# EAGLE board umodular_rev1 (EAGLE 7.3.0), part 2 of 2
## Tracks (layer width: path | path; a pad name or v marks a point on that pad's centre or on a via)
GND  (via drill 0.51)
  Top 0.356: 5K1.3 90.27,89.97 90.27,92.71 88.14,94.84 5K1.2 | 102.77,71.07 102.77,68.33 10K1.2 | 102.77,71.07 104.9,73.2 10K1.1 | 102.77,71.07 100.02,71.07 93.32,77.77 R18.P$1 | R15.P$2 82.96,84.18 86.92,84.18 93.02,78.08 R18.P$1 | TL274.10 75.95,40.89 77.77,42.72 77.77,43.94 75.95,45.77 TL274.12 | 10K.1 63.45,71.07 63.45,68.33 10K.2 63.14,68.33 61.01,66.19 61.01,65.28 64.06,62.23 64.06,50.04 68.02,46.08 TL274.3 | CA3046.4 75.95,63.45 77.77,63.45 82.65,68.33 R17.P$1 82.96,68.33 92.41,77.77 93.02,77.77 R18.P$1 | 197.87,69.85 198.48,69.85 199.39,70.76 DUALOPAMP.3 | 197.87,69.85 192.99,69.85 TL274-6.10 192.68,69.85 185.37,69.85 TL274-6.5 | 197.87,69.85 197.87,64.06 R99.P$1 | LM13700.13 161.9,83.26 165.25,83.26 166.17,84.18 C11.2 166.47,84.48 169.22,84.48 C10.2 | R56.P$1 175.31,87.22 178.66,83.87 181.1,83.87 R93.P$1 181.41,83.87 182.93,83.87 186.28,87.22 THAT2180.3 186.59,87.22 188.42,85.39 192.08,85.39 193.9,87.22 THAT2180.6 194.21,87.53 196.65,89.97 202.74,89.97 210.36,97.59 236.27,97.59 237.8,96.06 D1.A 238.1,95.76 239.32,94.54 241.45,94.54 244.5,91.49 | RES0NANCE.P$1 141.48,37.54 141.48,53.7 139.34,55.83 139.34,67.41 R48.P$2 139.04,67.72 139.04,69.24 135.99,72.29 135.99,78.08 | TL274-3.10 115.27,40.89 117.09,42.72 117.09,43.94 115.27,45.77 TL274-3.12 | R31.P$1 102.16,40.59 107.34,45.77 TL274-3.3 | CA3046-2.4 115.57,63.45 117.4,63.45 122.28,68.33 R40.P$1 122.58,68.33 132.33,78.08 | 5K3.3 129.9,89.97 129.9,92.41 127.46,94.84 5K3.2 | 135.99,78.08 132.64,78.08 R41.P$1 132.33,78.08 | R55.P$1 135.99,78.08 | 132.33,78.08 126.24,84.18 122.58,84.18 R38.P$2
  Top 0.356: U2.SLEEVE 368.86,17.12 368.86,18.03 372.52,21.69 372.52,43.64 368.86,47.3 U1.SLEEVE | 320.4,37.85 322.22,36.02 TL274-8.5 322.53,36.02 326.19,36.02 328.02,37.85 | 320.4,37.85 320.4,39.07 322.22,40.89 TL274-8.3 | 328.02,37.85 329.84,36.02 TL274-8.10 | 328.02,37.85 328.02,39.07 329.84,40.89 TL274-8.12 | 293.27,10.41 293.27,9.8 C17.1 | 293.27,10.41 289.92,13.77 ATT1.P$1 289.61,13.77 284.12,13.77 275.89,5.54 275.89,4.01 274.98,3.1 269.19,3.1 262.79,9.5 249.38,9.5 C14.1 249.07,9.8 244.5,14.38 ATT.P$1 244.5,14.68 244.5,17.73 251.82,25.04 251.82,33.27 C13.1 | 293.27,10.41 296.32,13.46 296.32,18.64 294.79,20.17 294.79,30.84 296.62,32.66 C16.1 296.93,32.97 301.8,37.85 320.4,37.85 | 555-1.1 288.7,86.31 288.7,96.06 287.17,97.59 284.43,97.59 282.9,96.06 D6.A 282.6,96.06 281.69,96.06 280.16,97.59 250.6,97.59 244.5,91.49 | 2N3904-4.1 276.2,70.46 276.2,75.95 2N3904-1.1 | v276.81,67.41 276.81,61.62 2N3904-5.1 | 244.5,91.49 244.5,86.61 | 244.5,86.61 244.5,86.31 555.1 244.5,86.61 | 2N3904.1 232,61.62 232,69.55 231.39,70.16 2N3904-2.1 231.39,70.46 231.39,74.42 | 231.39,74.42 231.39,75.95 2N3904-3.1 | 244.5,86.61 239.62,86.61 237.49,84.48 237.49,76.86 237.8,76.56 237.8,75.34 236.88,74.42 231.39,74.42
  Bottom 0.356: 5K1.3 90.58,89.66 90.58,80.52 93.02,78.08 R18.P$1 | R8.P$1 62.54,40.59 61.01,42.11 61.01,50.04 56.74,54.3 JP3.2 56.74,54.61 61.01,58.88 61.01,66.19 63.14,68.33 10K.2 | TL274.3 68.33,45.77 75.64,45.77 TL274.12 | 10K.1 65.89,73.2 68.33,73.2 73.81,67.72 73.81,65.58 75.95,63.45 CA3046.4 | TL274-6.5 185.37,69.85 187.2,71.68 187.2,72.9 185.37,74.73 TL274-6.3 | R56.P$1 175.01,87.22 172.26,87.22 169.52,84.48 C10.2 | DUALOPAMP.3 199.39,71.07 199.39,71.68 194.82,76.25 194.82,86.61 194.21,87.22 THAT2180.6 | TL274-3.12 114.96,45.77 107.64,45.77 TL274-3.3 107.34,46.08 105.51,47.9 105.51,51.26 108.56,54.3 108.86,54.3 113.44,58.88 113.44,61.32 115.27,63.14 CA3046-2.4 115.27,63.45 113.44,65.28 113.44,67.72 107.95,73.2 105.21,73.2 10K1.1 | R41.P$1 132.33,78.08 130.2,80.21 130.2,89.66 5K3.3 130.2,89.97 132.94,92.71 149.71,92.71 152.76,89.66 155.19,89.66 161.59,83.26 LM13700.13 | C16.1 296.62,32.97 296.62,36.02 292.35,40.28 292.35,48.51 289.31,51.56 D7.A | U2.SLEEVE 368.55,16.81 368.55,14.38 364.29,10.11 361.24,10.11 336.55,34.8 336.55,38.76 334.42,40.89 330.15,40.89 TL274-8.12 | v276.81,67.41 276.81,69.85 276.5,70.16 2N3904-4.1 | D6.A 282.6,95.76 282.6,93.02 276.5,86.92 276.5,76.25 2N3904-1.1 | 2N3904.1 232.31,61.62 242.06,51.87 D2.A 244.5,51.56 244.5,32.97 245.42,32.05 246.63,32.05 247.85,33.27 251.82,33.27 C13.1
  pour Bottom: 0.1,99.85 373.28,99.85 373.28,0 0.1,0
N$1
  Top 0.356: R6.P$2 R5.P$2 | R2.P$2 62.84,27.79 65.58,27.79 R3.P$2 65.89,27.79 68.94,27.79 R4.P$2
  Bottom 0.356: TL274.2 68.02,48.21 62.84,43.03 R1.P$1 62.84,42.72 62.84,42.11 65.58,39.37 65.58,27.79 R3.P$2 | R6.P$2 65.58,14.99 65.58,15.6 64.06,17.12 64.06,26.26 62.84,27.48 R2.P$2
N$2
  Bottom 0.356: R1.P$2 62.84,53.09 64.97,50.95 68.02,50.95 TL274.1 68.33,50.65 71.98,46.99 77.16,46.99 80.82,43.33 83.26,43.33 87.83,38.76 93.02,38.76 R7.P$2
N$3
  Top 0.356: CVS.5 79.6,21.08 66.19,21.08 62.84,17.73 R2.P$1
N$4
  Top 0.356: CVS.4 79.91,18.95 67.11,18.95 65.89,17.73 R3.P$1
N$5
  Top 0.356: CVS.3 79.6,16.51 70.16,16.51 69.24,17.42 R4.P$1
N$6
  Top 0.356: CVS.2 79.91,13.46 71.37,13.46 62.84,4.93 R5.P$1
N$7
  Top 0.356: R6.P$1 71.98,11.02 79.6,11.02 CVS.1
N$8
  Top 0.356: R7.P$1 82.96,38.46 82.96,31.75 83.57,31.14 5K.3
N$9
  Top 0.356: 5K.1 78.69,31.14 78.69,33.58 80.82,35.71 5K.2 | TL274.5 68.02,40.59 62.84,35.41 62.84,30.23 R8.P$2
  Bottom 0.356: 5K.1 78.38,31.14 77.77,31.14 68.33,40.59 TL274.5
N$10
  Top 0.356: TL274.7 68.33,35.71 68.33,38.15 TL274.6 68.33,38.46 70.16,40.28 70.16,52.17 75.95,57.96 CA3046.2
N$11
  Top 0.356: JP1.3 93.02,21.39 93.02,34.49 82.96,44.55 R11.P$1
N$12
  Top 0.356: TL274.8 75.95,35.71 78.38,38.15 78.38,48.51 79.6,49.73 C1.2 79.91,50.04 81.43,51.56 82.65,51.56 R10.P$1
N$13
  Top 0.356: CA3046.5 75.95,65.89 77.16,65.89 82.65,71.37 R12.P$1
N$14
  Top 0.356: CA3046.1 75.95,55.52 72.29,51.87 72.29,41.81 75.64,38.46 TL274.9 75.64,38.15 73.81,36.32 73.81,35.1 74.73,34.19 76.86,34.19 79.6,36.93 79.6,47.3 C1.1
  Bottom 0.356: 91.49,46.38 82.96,46.38 82.04,47.3 79.91,47.3 C1.1 | 91.49,46.38 93.02,44.86 R11.P$2 | 91.49,46.38 91.49,52.17 93.02,53.7 93.02,54.91 R9.P$1
N$15
  Top 0.356: CA3046.3 84.18,60.71 93.02,51.87 R10.P$2
N$16
  Top 0.356: C2.1 82.65,63.14 85.09,60.71 87.53,60.71 J112.2 87.83,60.71 87.83,65.28 93.02,70.46 93.02,71.37 R12.P$2
  Bottom 0.356: TL274.13 75.95,48.51 80.21,52.78 80.21,61.01 82.35,63.14 C2.1
N$17
  Top 0.356: C4.1 79.3,72.29 80.52,72.29 82.65,74.42 R13.P$1 | TL274.14 75.95,50.95 75.95,51.87 82.35,58.27 C2.2
  Bottom 0.356: C2.2 82.65,58.57 83.26,59.18 89.36,59.18 J112.3 89.66,59.49 90.88,60.71 90.88,65.58 82.96,73.51 82.96,74.42 R13.P$1
N$18
  Top 0.356: TL274-2.10 68.02,86 65.28,86 64.67,86.61 R20.P$2
N$19
  Top 0.356: C3.2 78.99,77.16 77.47,77.16 75.95,75.64 TL274-2.1
  Bottom 0.356: J112.1 89.36,62.23 86.92,62.23 75.95,73.2 75.95,75.34 TL274-2.1
N$20
  Top 0.356: TL274-2.9 68.33,88.14 73.81,82.65 73.81,60.4 74.73,59.49 81.43,59.49 81.74,59.79 82.96,59.79 93.02,49.73 93.02,48.82 R21.P$1
N$21
  Top 0.356: R15.P$1 93.32,84.18 93.32,81.13 R14.P$2
  Bottom 0.356: TL274-2.2 75.95,78.08 78.08,75.95 82.04,75.95 82.35,76.25 89.36,76.25 92.41,73.2 93.62,73.2 94.54,74.12 94.54,79.6 93.32,80.82 R14.P$2
N$22
  Top 0.356: JP1.1 93.02,16.51 85.09,24.43 85.09,41.5 83.26,43.33 82.35,43.33 81.43,44.25 81.43,47.3 82.65,48.51 R21.P$2
N$23
  Top 0.356: TL274-2.3 75.95,80.52 78.38,80.52 78.99,79.91 C3.1 | 93.32,68.33 94.54,67.11 94.54,44.25 93.32,43.03 93.32,41.81 R16.P$1 | 93.32,68.33 94.54,69.55 94.54,72.29 93.32,73.51 93.32,74.42 R13.P$2 | 93.32,68.33 R17.P$2
  Bottom 0.356: C3.1 79.3,79.6 88.14,79.6 93.02,74.73 R13.P$2
N$24
  Bottom 0.356: JP1.2 93.32,18.95 92.71,18.95 85.09,26.57 85.09,39.37 82.96,41.5 R16.P$2
N$25
  Top 0.356: 82.65,78.08 82.65,78.99 75.95,85.7 TL274-2.5 | 82.65,78.08 79.3,74.73 C4.2 | 82.65,78.08 R18.P$2
N$26
  Top 0.356: TL274-2.6 75.95,88.44 82.04,88.44 83.26,89.66 85.39,89.66 5K1.1 85.7,89.66 87.83,87.53 93.02,87.53 R19.P$1
N$27
  Top 0.356: JP2.2 93.02,7.06 93.02,10.72 77.47,26.26 61.93,26.26 53.39,34.8 53.39,64.06 64.36,75.03 64.36,76.56 R20.P$1
  Bottom 0.356: R19.P$2 82.65,87.53 79.6,90.58 75.95,90.58 TL274-2.7 75.64,90.58 69.55,84.48 66.8,84.48 64.67,82.35 64.67,76.86 R20.P$1
N$28
  Top 0.356: TL274-2.8 68.02,90.58 61.62,90.58 R22.P$1
N$29
  Top 0.356: R22.P$2 61.32,80.21 61.32,74.12 60.71,73.51 10K.3
  Bottom 0.356: JP2.1 93.02,4.32 92.1,4.32 81.43,14.99 76.25,14.99 64.06,27.18 64.06,36.93 54,46.99 54,66.5 60.71,73.2 10K.3
N$30
  Top 0.356: TL274-3.2 107.34,48.21 102.16,43.03 R24.P$1 | R29.P$2 R28.P$2 | R25.P$2 102.16,27.79 104.9,27.79 R26.P$2 105.21,27.79 108.25,27.79 R27.P$2
  Bottom 0.356: R29.P$2 104.9,14.99 104.9,15.6 103.38,17.12 103.38,26.26 102.16,27.48 R25.P$2 | R24.P$1 102.16,42.72 104.9,39.98 104.9,27.79 R26.P$2
N$31
  Top 0.356: CA3046.14 CA3046.13 CA3046.12 63.45,65.58 62.84,65.58 R23.P$2
N$32
  Top 0.356: TL274-3.1 107.34,50.95 104.29,50.95 102.16,53.09 R24.P$2
  Bottom 0.356: R30.P$2 132.33,38.76 127.15,38.76 122.58,43.33 120.14,43.33 116.48,46.99 111.3,46.99 107.64,50.65 TL274-3.1
N$33
  Top 0.356: CVS1.5 118.92,21.08 105.51,21.08 102.16,17.73 R25.P$1
N$34
  Top 0.356: CVS1.4 119.23,18.95 106.43,18.95 105.21,17.73 R26.P$1
N$35
  Top 0.356: CVS1.3 118.92,16.51 109.47,16.51 108.56,17.42 R27.P$1
N$36
  Top 0.356: CVS1.2 119.23,13.46 110.69,13.46 102.16,4.93 R28.P$1
N$37
  Top 0.356: CVS1.1 118.92,11.02 111.3,11.02 105.21,4.93 R29.P$1
N$38
  Top 0.356: R30.P$1 122.58,38.46 122.58,31.45 122.88,31.14 5K2.3
N$39
  Top 0.356: 5K2.1 118.01,31.14 118.01,33.58 120.14,35.71 5K2.2 | TL274-3.5 107.34,40.59 102.16,35.41 102.16,30.23 R31.P$2
  Bottom 0.356: 5K2.1 117.7,31.14 117.09,31.14 107.64,40.59 TL274-3.5
N$40
  Top 0.356: 107.64,38.15 107.64,35.71 TL274-3.7 | 107.64,38.15 109.47,39.98 109.47,52.17 115.27,57.96 CA3046-2.2 | 107.64,38.15 TL274-3.6
N$41
  Top 0.356: TL274-3.8 115.27,35.71 117.7,38.15 117.7,48.51 118.92,49.73 C5.2 119.23,50.04 120.75,51.56 122.28,51.56 R33.P$1
N$42
  Top 0.356: 113.74,38.46 114.96,38.46 TL274-3.9 | 113.74,38.46 110.39,41.81 110.39,50.65 115.27,55.52 CA3046-2.1 | R34.P$2 132.33,44.86 130.81,46.38 122.58,46.38 121.67,47.3 119.23,47.3 C5.1 118.92,47.3 118.92,36.93 116.18,34.19 114.05,34.19 113.13,35.1 113.13,36.02 113.74,36.63 113.74,38.46
  Bottom 0.356: R32.P$1 132.64,54.91 132.64,53.7 133.86,52.48 133.86,46.08 132.64,44.86 R34.P$2
N$43
  Top 0.356: CA3046-2.3 123.49,60.71 132.33,51.87 R33.P$2
N$44
  Top 0.356: R34.P$1 132.33,34.8 132.33,21.39 JP4.3
N$45
  Top 0.356: CA3046-2.5 115.57,65.89 116.79,65.89 122.28,71.37 R35.P$1
N$46
  Top 0.356: C6.1 121.97,63.14 124.41,60.71 126.85,60.71 Q2.2 127.15,60.71 127.15,64.97 132.33,70.16 132.33,71.37 R35.P$2
  Bottom 0.356: TL274-3.13 115.27,48.51 119.84,53.09 119.84,61.32 121.67,63.14 C6.1
N$47
  Top 0.356: C8.1 118.62,72.29 120.14,72.29 122.28,74.42 R36.P$1 | TL274-3.14 115.27,50.95 115.27,51.87 121.67,58.27 C6.2
  Bottom 0.356: C6.2 121.97,58.57 122.58,59.18 128.68,59.18 Q2.3 128.98,59.49 130.2,60.71 130.2,65.58 122.58,73.2 122.58,74.42 R36.P$1
N$48
  Top 0.356: TL274-4.1 115.27,75.64 116.79,75.64 118.31,77.16 C7.2
  Bottom 0.356: Q2.1 128.68,62.23 126.24,62.23 117.4,71.07 117.4,71.37 115.27,73.51 115.27,75.34 TL274-4.1
N$49
  Top 0.356: R38.P$1 132.64,84.18 132.64,81.13 R37.P$2
  Bottom 0.356: TL274-4.2 115.27,78.08 117.4,75.95 121.36,75.95 121.67,76.25 128.68,76.25 131.72,73.2 132.94,73.2 133.86,74.12 133.86,79.6 132.64,80.82 R37.P$2
N$50
  Top 0.356: TL274-4.3 115.27,80.52 117.7,80.52 118.31,79.91 C7.1 | 132.64,68.33 133.86,67.11 133.86,44.25 132.64,43.03 132.64,41.81 R39.P$1 | 132.64,68.33 133.86,69.55 133.86,72.29 132.64,73.51 132.64,74.42 R36.P$2 | 132.64,68.33 R40.P$2
  Bottom 0.356: C7.1 118.62,79.6 127.46,79.6 132.33,74.73 R36.P$2
N$51
  Top 0.356: JP4.2 132.64,18.95 132.03,18.95 124.41,26.57 124.41,39.68 122.58,41.5 R39.P$2
N$52
  Top 0.356: TL274-4.5 115.27,85.7 122.28,78.69 122.28,78.08 R41.P$2 122.28,77.77 119.23,74.73 118.62,74.73 C8.2
N$53
  Top 0.356: TL274-4.6 115.27,88.44 121.36,88.44 122.58,89.66 124.71,89.66 5K3.1 125.02,89.66 127.15,87.53 132.33,87.53 R42.P$1
N$54
  Bottom 0.356: R42.P$2 122.28,87.53 119.23,90.58 115.27,90.58 TL274-4.7 114.96,90.58 108.86,84.48 106.43,84.48 103.99,82.04 103.99,76.86 R43.P$1 103.68,76.56 103.68,75.03 100.33,71.68 100.33,49.73 105.51,44.55 105.51,37.85 106.43,36.93 108.86,36.93 132.33,13.46 132.33,7.06 JP5.2
N$55
  Top 0.356: TL274-4.10 107.34,86 104.6,86 103.99,86.61 R43.P$2
N$56
  Top 0.356: TL274-4.9 107.64,88.14 113.13,82.65 113.13,60.4 114.05,59.49 121.06,59.49 121.36,59.79 122.28,59.79 132.33,49.73 132.33,48.82 R44.P$1
N$57
  Bottom 0.356: JP4.1 132.64,16.51 133.25,16.51 134.77,18.03 134.77,38.15 132.64,40.28 130.81,40.28 122.58,48.51 R44.P$2
N$58
  Top 0.356: TL274-4.8 107.34,90.58 100.94,90.58 R45.P$1
N$59
  Top 0.356: R45.P$2 100.63,80.21 100.63,73.81 100.33,73.51 10K1.3
  Bottom 0.356: JP5.1 132.33,4.32 131.42,4.32 120.75,14.99 115.88,14.99 103.38,27.48 103.38,36.93 99.72,40.59 99.72,72.9 100.02,73.2 10K1.3
N$60
  Top 0.356: CA3046-2.14 107.64,55.83 107.64,57.96 CA3046-2.13 107.64,58.27 107.64,60.71 | 107.64,60.71 102.77,65.58 102.16,65.58 R46.P$2 | 107.64,60.71 CA3046-2.12
N$61
  Top 0.356: C12.2 146.36,63.75 146.36,56.13 145.75,55.52 JP6.1
N$62
  Top 0.356: C12.1 141.48,64.06 141.48,82.04 139.34,84.18 R47.P$1
N$63
  Top 0.356: 156.11,77.47 154.28,75.64 LM13700.7 | 156.11,77.47 156.11,78.69 154.28,80.52 LM13700.5 | 156.11,77.47 156.72,76.86 162.81,76.86 163.73,77.77 163.73,79.3 164.34,79.91 166.17,79.91 168,81.74 169.22,81.74 C10.1
N$64
  Top 0.356: R54.P$1 164.95,78.38 164.95,77.16 163.73,75.95 163.73,75.03 163.12,74.42 159.77,74.42 153.06,67.72 149.4,67.72 R48.P$1
  Bottom 0.356: LM13700.3 153.98,85.7 150.62,85.7 149.4,84.48 R47.P$2 149.4,84.18 150.93,82.65 150.93,70.46 149.4,68.94 149.4,67.72 R48.P$1
N$65
  Top 0.356: LM13700.8 153.98,73.2 150.93,76.25 150.93,78.38 149.4,79.91 146.96,79.91 139.34,87.53 R51.P$2 | JP7.1 174.09,55.22 172.26,53.39 172.26,39.98 174.4,37.85 174.4,36.93 173.18,35.71 148.18,35.71 146.66,37.24 RES0NANCE.P$3 146.36,37.54 146.36,49.73 140.26,55.83 140.26,64.67 140.56,64.97 140.56,75.34 139.34,76.56 139.34,77.77 R50.P$2
  Bottom 0.356: 140.56,86.31 140.56,80.52 139.34,79.3 139.34,78.08 R50.P$2 | 140.56,86.31 139.34,87.53 R51.P$2 | 140.56,86.31 145.14,90.88 149.1,90.88 R49.P$1
N$66
  Top 0.356: R56.P$2 164.95,87.22 163.73,86 161.9,86 LM13700.14 161.59,86 157.94,89.66 148.79,89.66 147.57,90.88 139.34,90.88 R49.P$2
N$67
  Top 0.356: 150.93,82.96 153.98,82.96 LM13700.4 | 150.93,82.96 149.4,81.43 R55.P$2 | 150.93,82.96 150.93,85.09 149.4,86.61 149.4,87.53 R51.P$1
  Bottom 0.356: R53.P$1 149.1,74.73 149.1,76.25 147.88,77.47 147.88,79.91 149.1,81.13 R55.P$2
N$68
  Top 0.356: R53.P$2 139.34,74.42 139.34,71.37 R52.P$2
  Bottom 0.356: R52.P$2 139.34,71.07 141.48,71.07 147.88,64.67 153.37,64.67 161.59,72.9 LM13700.9 161.9,73.2 162.2,73.51 165.25,73.51 166.47,74.73 166.47,79.3 164.95,80.82 164.95,85.09 172.26,92.41 175.62,92.41 176.84,91.19 176.84,54.91 JP7.2
N$69
  Top 0.356: C11.1 166.17,81.74 162.81,81.74 161.9,80.82 LM13700.12
  Bottom 0.356: LM13700.10 161.59,75.64 159.77,77.47 159.77,78.69 161.59,80.52 LM13700.12
N$70
  Top 0.356: R61.P$2 162.81,71.68 164.95,73.81 164.95,75.03 R58.P$1 | LM13700.1 154.28,90.88 161.59,90.88 LM13700.16 161.9,90.88 164.95,90.88 R57.P$1
  Bottom 0.356: R58.P$1 164.95,75.34 164.95,76.56 163.73,77.77 163.73,89.36 164.95,90.58 R57.P$1
N$71
  Bottom 0.356: RES0NANCE.P$2 143.92,37.54 144.53,37.54 157.63,50.65 157.63,53.09 158.55,54 160.99,54 173.18,66.19 173.18,76.56 175.01,78.38 R54.P$2
N$72
  Bottom 0.356: JP8.2 160.07,55.52 160.07,61.32 168,69.24 168,85.09 173.48,90.58 175.01,90.58 R57.P$2
N$73
  Bottom 0.356: JP8.1 160.07,52.78 160.68,52.78 173.79,65.89 173.79,73.81 175.01,75.03 R58.P$2
N$74
  Bottom 0.356: CUTOFF.P$1 168,37.54 168,59.18 175.01,66.19 175.01,71.98 R60.P$2
N$75
  Top 0.356: R59.P$2 162.81,50.04 171.65,41.2 171.65,38.46 172.57,37.54 CUTOFF.P$3
N$76
  Top 0.356: R61.P$1 152.45,69.24 148.79,69.24 147.88,68.33 147.88,59.18 168.3,38.76 168.91,38.76 170.13,37.54 CUTOFF.P$2
N$77
  Top 0.356: TRIG_IN.1 221.34,22 221.34,16.51 S1.1
  Bottom 0.356: R62.P$1 251.82,95.76 243.59,95.76 241.45,93.62 232.31,93.62 228.96,90.27 227.43,90.27 214.94,77.77 214.94,28.7 221.34,22.3 TRIG_IN.1
N$78
  Top 0.356: 2N3904-3.2 233.53,76.25 233.53,92.71 230.48,95.76 D1.C
  Bottom 0.356: D1.C 230.48,95.76 235.97,95.76 237.19,94.54 240.23,94.54 241.45,95.76 R62.P$2
N$79
  Top 0.356: 555.2 244.5,83.87 241.45,83.87 240.23,85.09 R67.P$1
  Bottom 0.356: 2N3904.3 237.19,61.62 237.19,69.24 240.54,72.59 240.54,84.78 240.23,85.09 R67.P$1
N$80
  Top 0.356: 555.4 244.5,78.38 236.58,70.46 2N3904-2.3 | C9.1 251.82,42.72 251.21,42.72 240.54,32.05 239.32,32.05 237.8,33.58 237.8,47.6 239.62,49.43 R70.P$1
  Bottom 0.356: R65.P$1 239.01,88.44 242.67,84.78 242.67,80.52 244.5,78.69 555.4 | 2N3904-2.3 236.27,70.16 236.27,68.02 230.48,62.23 230.48,59.18 239.93,49.73 R70.P$1
N$81
  Top 0.356: 2N3904-3.3 236.58,76.25 236.58,89.97 238.71,92.1 R63.P$1 239.01,92.41 241.45,92.41 R64.P$1
N$82
  Top 0.356: 2N3904-2.2 233.83,70.46 243.28,79.91 246.02,79.91 250.29,84.18 250.29,90.58 251.82,92.1 R64.P$2
N$83
  Top 0.356: D2.C 251.82,51.56 251.82,48.21 C9.2 251.82,47.9 247.55,43.64 246.02,43.64 R66.P$1
N$84
  Bottom 0.356: 2N3904.2 234.75,61.32 237.19,58.88 239.93,58.88 247.55,51.26 247.55,35.1 246.02,33.58 R66.P$2
N$85
  Top 0.356: TL274-5.3 244.5,66.8 243.59,65.89 243.28,65.89 239.32,61.93 239.32,59.49 232.92,53.09 232.92,52.78 231.09,50.95 228.96,50.95 225.6,47.6 225.6,47.3 224.69,46.38 223.16,46.38 221.64,47.9 SUSTAIN.P$2
N$86
  Bottom 0.356: 555.5 252.12,78.38 252.12,74.73 250.29,72.9 250.29,40.28 251.82,38.76 C13.2
N$87
  Top 0.356: 555.7 252.12,83.57 237.8,69.24 237.8,62.84 238.71,61.93 238.71,59.79 232.31,53.39 232.31,53.09 230.78,51.56 227.74,51.56 224.38,48.21 SUSTAIN.P$3
N$88
  Bottom 0.356: SUSTAIN.P$1 219.2,48.21 219.2,50.95 225.6,57.35 228.96,57.35 R68.P$1
N$89
  Top 0.356: TL274-5.1 244.5,71.98 244.5,69.85 TL274-5.2 244.5,69.55 242.67,69.55 239.62,66.5 R69.P$1
N$90
  Top 0.356: DECAY.P$1 219.2,63.75 221.34,63.75 DECAY.P$2 221.64,63.75 224.08,66.19 228.96,66.19 R69.P$2
N$91
  Top 0.356: DECAY.P$3 224.38,63.45 224.38,59.79 230.48,53.7 D3.C
N$92
  Top 0.356: C14.2 244.2,9.8 237.19,9.8 D5.C 237.19,9.5 237.19,4.62 D4.A | D3.A 238.4,53.7 240.84,56.13 240.84,58.27 244.5,61.93 TL274-5.5 244.81,62.23 246.63,64.06 246.63,75.34 252.12,80.82 555.6
  Bottom 0.356: D5.C 237.19,9.8 237.19,14.68 239.93,17.42 239.93,31.45 241.45,32.97 241.45,50.34 238.4,53.39 D3.A
N$93
  Top 0.356: 555.3 244.5,81.13 239.32,81.13 239.01,81.43 R71.P$1
N$94
  Top 0.356: ATTACK.P$1 219.2,79.3 221.34,79.3 ATTACK.P$2 221.64,79.3 223.77,81.43 228.65,81.43 R71.P$2
N$95
  Top 0.356: RELEASE.P$1 219.2,32.05 221.34,32.05 RELEASE.P$2 221.64,32.36 221.64,39.68 229.56,47.6 229.56,49.43 R70.P$2
N$96
  Top 0.356: D4.C 229.26,4.62 229.26,7.67 224.38,12.55 224.38,32.05 RELEASE.P$3
N$97
  Bottom 0.356: D5.A 229.26,9.8 229.26,32.05 228.35,32.97 228.35,54.61 230.78,57.05 230.78,57.96 225.6,63.14 225.6,68.33 224.08,69.85 224.08,78.99 ATTACK.P$3
N$98
  Top 0.356: TL274-5.6 244.5,59.18 244.5,57.05 TL274-5.7 244.5,56.74 244.5,55.22 242.06,52.78 242.06,47.9 239.93,45.77 R72.P$1
N$99
  Top 0.356: ATT.P$2 246.94,14.68 249.07,14.68 ATT.P$3 | TL274-5.10 252.12,61.93 242.67,52.48 242.67,46.38 240.54,44.25 239.32,44.25 238.4,45.16 238.4,46.38 239.93,47.9 240.23,47.9 241.45,49.12 241.45,50.04 240.54,50.95 235.05,50.95 229.87,45.77 R72.P$2
  Bottom 0.356: ATT.P$3 249.38,14.68 249.38,29.01 254.25,33.88 254.25,60.1 252.43,61.93 TL274-5.10
N$100
  Top 0.356: R75.P$1 239.93,33.58 239.93,37.24 R74.P$1 239.93,37.54 239.93,41.2 R73.P$1 239.93,41.5 239.93,42.11 252.12,54.3 252.12,56.74 TL274-5.8 252.12,57.05 252.12,59.18 TL274-5.9
N$101
  Top 0.356: JP9.1 236.58,22 236.58,34.49 229.87,41.2 R73.P$2
N$102
  Top 0.356: JP9.2 236.27,19.56 231.39,24.43 231.39,35.71 229.87,37.24 R74.P$2
N$103
  Top 0.356: JP9.3 235.36,18.03 235.05,18.03 229.87,23.22 229.87,33.27 R75.P$2
N$104
  Top 0.356: TRIG_IN1.1 266.75,22 266.75,16.81 266.45,16.51 S2.1
  Bottom 0.356: R76.P$1 296.62,96.06 288.7,96.06 287.17,97.59 281.08,97.59 273.76,90.27 272.24,90.27 259.13,77.16 259.13,29.92 266.75,22.3 TRIG_IN1.1
N$105
  Top 0.356: 278.94,95.76 281.08,95.76 282.3,94.54 285.34,94.54 286.56,95.76 R76.P$2 | 278.94,95.76 275.28,95.76 D6.C | 278.94,95.76 278.94,76.25 2N3904-1.2
N$106
  Top 0.356: 555-1.2 288.7,83.87 285.34,83.87 284.12,85.09 R81.P$1
  Bottom 0.356: 2N3904-5.3 282.3,61.62 282.3,68.33 286.87,72.9 286.87,81.74 288.7,83.57 555-1.2
N$107
  Top 0.356: 287.17,76.25 281.38,70.46 2N3904-4.3 | 287.17,76.25 288.7,77.77 288.7,78.38 555-1.4 | 287.17,76.25 282.3,81.13 282.3,85.7 283.82,87.22 283.82,88.44 R79.P$1
  Bottom 0.356: R84.P$1 285.04,48.82 286.26,47.6 286.26,35.41 290.52,31.14 296.93,31.14 298.14,32.36 298.14,38.46 296.93,39.68 296.93,42.11 C15.1 296.62,42.42 295.4,43.64 295.4,47.6 289.61,53.39 285.04,53.39 282.9,55.52 282.9,56.74 283.51,57.35 283.51,61.62 287.78,65.89 290.22,65.89 290.83,66.5 290.83,72.59 289,74.42 289,78.38 555-1.4
N$108
  Top 0.356: 2N3904-1.3 281.38,76.25 281.38,89.66 283.82,92.1 R77.P$1 284.12,92.41 286.56,92.41 R78.P$1
N$109
  Bottom 0.356: 2N3904-4.2 278.94,70.46 278.94,71.68 285.65,78.38 285.65,85.39 292.35,92.1 296.62,92.1 R78.P$2
N$110
  Top 0.356: D7.C 296.93,51.56 296.93,47.6 C15.2 296.62,47.3 292.35,43.03 291.13,43.03 R80.P$1
N$111
  Bottom 0.356: 2N3904-5.2 279.55,61.32 279.55,57.96 289.31,48.21 289.31,34.49 290.83,32.97 R80.P$2
N$112
  Top 0.356: 555-1.5 296.62,78.38 296.62,74.42 298.45,72.59 298.45,39.68 296.93,38.15 C16.2
N$113
  Bottom 0.356: 555-1.7 296.32,83.87 291.13,83.87 290.22,84.78 287.48,84.78 286.26,83.57 286.26,73.2 268.88,55.83 268.88,48.21 SUSTAIN1.P$3
N$114
  Top 0.356: SUSTAIN1.P$1 264.01,48.21 264.62,48.21 269.19,52.78 271.63,52.78 274.07,55.22 274.07,56.13 R82.P$1
N$115
  Top 0.356: TL274-1.3 288.7,66.8 285.95,64.06 285.95,55.83 283.82,53.7 279.25,53.7 275.89,50.34 268.58,50.34 266.45,48.21 SUSTAIN1.P$2
N$116
  Top 0.356: TL274-1.1 289,71.98 289,69.85 TL274-1.2 288.7,69.55 287.48,69.55 284.43,66.5 R83.P$1
N$117
  Top 0.356: DECAY1.P$1 264.01,63.75 266.14,63.75 DECAY1.P$2 266.45,63.75 268.88,66.19 274.07,66.19 R83.P$2
N$118
  Top 0.356: DECAY1.P$3 268.88,63.45 275.59,56.74 275.59,52.48 D8.C
N$119
  Top 0.356: C17.2 288.39,9.8 282.3,9.8 D10.C 282.3,9.5 282.3,4.62 D9.A | D8.A 283.51,52.48 286.56,55.52 286.56,59.79 288.7,61.93 TL274-1.5 289,62.23 290.83,64.06 290.83,75.34 296.32,80.82 555-1.6
  Bottom 0.356: D10.C 282.3,9.8 282.3,14.07 284.43,16.2 284.43,31.75 283.21,32.97 283.21,52.17 D8.A
N$120
  Top 0.356: RELEASE1.P$1 264.01,32.05 266.14,32.05 RELEASE1.P$2 266.45,32.36 266.45,38.76 274.68,46.99 274.68,48.82 R84.P$2
N$121
  Top 0.356: RELEASE1.P$3 268.88,32.05 268.88,23.22 272.85,19.25 272.85,6.15 274.37,4.62 D9.C
N$122
  Top 0.356: 555-1.3 288.7,81.13 284.43,81.13 284.12,81.43 R85.P$1
N$123
  Top 0.356: ATTACK1.P$1 264.01,79.3 266.14,79.3 ATTACK1.P$2 266.45,79.3 268.58,81.43 273.46,81.43 R85.P$2
N$124
  Bottom 0.356: ATTACK1.P$3 268.58,78.99 268.58,70.46 259.74,61.62 259.74,32.36 274.37,17.73 274.37,9.8 D10.A
N$125
  Top 0.356: TL274-1.6 289,59.18 289,57.05 TL274-1.7 288.7,56.74 288.7,55.22 286.26,52.78 286.26,46.38 285.04,45.16 R86.P$1
N$126
  Top 0.356: ATT1.P$3 294.79,14.07 292.35,14.07 ATT1.P$2 292.05,14.07 292.05,24.13 283.21,32.97 283.21,43.33 | 283.21,43.33 276.5,43.33 274.98,44.86 R86.P$2 | 283.21,43.33 285.34,43.33 286.87,44.86 286.87,52.48 296.32,61.93 TL274-1.10
N$127
  Top 0.356: R89.P$1 285.04,33.58 285.04,37.24 R88.P$1 285.04,37.54 285.04,41.2 R87.P$1 285.04,41.5 285.04,42.11 296.32,53.39 296.32,56.74 TL274-1.8 296.62,57.05 296.62,59.18 TL274-1.9
N$128
  Top 0.356: JP10.1 281.99,22 281.99,34.19 274.98,41.2 R87.P$2
N$129
  Top 0.356: JP10.2 281.69,19.56 276.2,25.04 276.2,36.02 274.98,37.24 R88.P$2
N$130
  Top 0.356: JP10.3 281.99,16.81 280.77,18.03 280.47,18.03 274.98,23.52 274.98,33.27 R89.P$2
N$131
  Top 0.356: R91.P$2 203.05,30.23 203.05,27.18 R92.P$2 203.05,26.87 206.4,26.87 R90.P$1
  Bottom 0.356: TL274-6.2 185.37,77.16 189.33,73.2 189.33,43.33 202.13,30.53 202.74,30.53 R91.P$2
N$132
  Top 0.356: TL274-6.1 185.37,80.21 185.37,83.26 D11.A
  Bottom 0.356: R90.P$2 206.4,36.93 206.4,31.75 203.35,28.7 202.44,28.7 188.42,42.72 188.42,58.88 183.24,64.06 183.24,78.08 185.06,79.91 TL274-6.1
N$133
  Top 0.356: JP11.2 188.72,30.53 192.68,30.53 R91.P$1
N$134
  Top 0.356: JP11.1 188.72,27.48 192.38,27.48 192.68,27.18 R92.P$1
N$135
  Top 0.356: R94.P$2 181.41,60.4 181.41,63.45 185.06,67.11 TL274-6.6 185.37,67.11 192.99,59.49 193.9,59.49 R95.P$1
N$136
  Top 0.356: 10K-2.1 180.8,50.95 180.8,53.39 183.24,55.83 10K-2.2 183.54,56.13 183.84,56.44 183.84,59.18 R95.P$2
N$137
  Top 0.356: R94.P$1 181.41,70.46 181.41,73.51 R93.P$2 181.41,73.81 181.41,75.95 184.15,78.69 186.59,78.69 191.16,83.26 192.68,83.26 D11.C
N$138
  Top 0.356: TL274-6.7 185.37,64.67 185.37,51.26 185.67,50.95 10K-2.3 185.98,50.95 186.59,51.56 197.26,51.56 R96.P$1
N$139
  Top 0.356: 206.4,55.83 206.4,58.57 207.62,59.79 R97.P$1 | 206.4,55.83 206.4,54.91 207.62,53.7 207.62,51.87 R96.P$2 | 206.4,55.83 197.87,55.83 R100.P$2
  Bottom 0.356: TL274-6.9 192.99,67.11 196.04,64.06 196.04,57.35 197.56,55.83 R100.P$2
N$140
  Top 0.356: TL274-6.8 192.99,64.67 197.56,60.1 R97.P$2
  Bottom 0.356: THAT2180.2 184.15,87.22 184.15,86.61 189.94,80.82 189.94,67.72 192.68,64.97 TL274-6.8
N$141
  Top 0.356: TL274-6.12 192.99,75.03 194.82,75.03 201.83,82.04 500.2 202.13,82.35 204.27,84.48 206.71,84.48 500.3 206.71,84.78 206.71,91.19 R98.P$1
N$142
  Bottom 0.356: 500.1 207.01,79.6 207.01,78.38 208.53,76.86 208.53,64.67 207.92,64.06 R99.P$2
N$143
  Top 0.356: TL274-6.13 192.99,77.47 192.99,79.91 TL274-6.14
  Bottom 0.356: TL274-6.13 192.99,77.16 198.17,71.98 198.17,65.58 207.92,55.83 R100.P$1
N$144
  Top 0.356: THAT2180.5 191.47,87.53 187.81,91.19 182.63,91.19 R101.P$2
N$145
  Top 0.356: C18.1 182.32,42.72 182.32,40.28 188.42,34.19 AUDIO_IN.1
N$146
  Top 0.356: C18.2 187.2,43.03 191.47,47.3 R102.P$1
N$147
  Bottom 0.356: THAT2180.1 181.1,87.22 181.1,85.39 179.27,83.57 179.27,49.43 181.1,47.6 R102.P$2
N$148
  Top 0.356: C19.1 201.83,47.6 197.56,43.33 R103.P$1
  Bottom 0.356: THAT2180.8 199.09,87.22 199.09,77.77 198.17,76.86 198.17,75.03 199.39,73.81 DUALOPAMP.2 199.7,73.51 200.91,72.29 200.91,64.67 209.45,56.13 209.45,55.22 208.23,54 207.92,54 206.1,52.17 206.1,51.87 202.13,47.9 C19.1
N$149
  Top 0.356: C19.2 204.57,47.6 204.57,46.38 207.62,43.33 R103.P$2 207.62,43.03 202.13,37.54 202.13,33.88 AUDIO_OUT.1
  Bottom 0.356: DUALOPAMP.1 199.7,75.95 199.7,75.34 205.79,69.24 205.79,64.06 210.06,59.79 210.06,51.87 206.1,47.9 204.57,47.9 C19.2
N$150
  Top 0.356: D12.A 49.12,45.47 49.12,49.12 D13.C 48.82,49.43 48.82,51.56 47.3,53.09 47.3,58.57 50.34,61.62 50.34,70.76 35.1,86 29.92,86 J1.PWR
N$151
  Top 0.356: 18.34,25.65 18.34,26.57 C27.1 | 18.34,25.65 18.34,10.72 C20.1 | 18.34,25.65 27.79,25.65 29.01,26.87 32.05,26.87 C22.1 | LM7809.IN 27.79,62.54 21.08,62.54 18.03,59.49 C21.1 | D14.C 49.12,57.66 49.12,55.52 50.34,54.3 50.34,44.55 49.43,43.64 40.28,43.64 38.76,45.16 D12.C
  Bottom 0.356: D12.C 38.46,45.47 38.46,46.69 28.09,57.05 28.09,62.54 LM7809.IN | C27.1 18.03,26.87 18.03,41.5 16.81,42.72 16.81,58.27 17.73,59.18 C21.1
N$152
  Top 0.356: C20.2 8.89,10.72 8.89,26.57 C27.2 8.89,26.87 8.89,36.32 | C21.2 8.59,59.18 8.59,43.33 C23.2 8.89,43.03 8.89,36.32 | J1.GND 29.62,93.32 25.96,89.66 J1.GNDBREAK | JP13.2 40.28,18.03 40.28,22.91 JP12.2 | 27.18,36.32 27.18,27.18 C22.2 | LM7809.GND 30.53,62.54 30.53,58.57 27.18,55.22 C28.2 27.18,54.91 27.18,45.77 C29.2 27.18,45.47 27.18,36.32 | 27.18,36.32 C25.2 8.89,36.32 | 30.84,63.14 30.53,62.84 LM7809.GND | 30.84,63.14 33.88,66.19 38.46,66.19 R105.P$2 | 30.84,63.14 18.64,75.34 17.73,75.34 C26.2 | 30.84,63.14 LM7809.GND
  Bottom 0.356: 19.25,82.65 25.96,89.36 J1.GNDBREAK | 19.25,82.65 17.73,81.13 17.73,75.64 C26.2 | 19.25,82.65 8.89,93.02 C24.2 | 48.82,40.89 48.82,43.03 47.3,44.55 47.3,51.87 48.82,53.39 D16.A | 47.6,23.22 45.16,23.22 43.33,25.04 42.11,25.04 40.28,23.22 JP12.2 39.98,23.22 37.54,25.65 28.4,25.65 27.18,26.87 C22.2 | LM7909.GND 43.94,71.37 38.76,66.19 R105.P$2 | 48.82,40.89 48.82,38.46 47.6,37.24 47.6,23.22 | 48.82,40.89 D17.C | 47.6,23.22 LED1.K
N$153
  Top 0.356: C26.1 8.28,75.64 8.28,83.26 18.03,93.02 C24.1 18.34,93.02 39.68,71.68 41.5,71.68 LM7909.IN 41.5,71.37 41.5,52.17 38.76,49.43 D13.A 38.46,49.12 38.46,46.99 37.24,45.77 37.24,38.15 38.76,36.63 D15.A
  Bottom 0.356: D15.A 38.76,36.32 C25.1 32.05,36.32 25.35,43.03 18.34,43.03 C23.1
N$154
  Bottom 0.356: TL274-7.3 342.95,60.4 339.9,57.35 326.8,57.35 324.97,59.18 324.97,59.49 317.04,67.41 311.56,67.41 309.73,69.24 309.73,70.16 307.29,72.59 RV1.P$2
N$155
  Top 0.356: LM7809.OUT 33.27,62.54 38.15,62.54 38.46,62.23 R104.P$1 38.76,62.23 38.76,57.96 D14.A 38.46,57.66 38.46,56.13 37.24,54.91 | JP13.3 37.85,17.73 37.85,22.61 JP12.3 37.54,22.91 37.54,36.93 36.63,37.85 36.63,51.56 38.46,53.39 D16.C 38.46,53.7 37.24,54.91 | 37.24,54.91 32.36,54.91 C28.1
N$156
  Top 0.356: LM7909.OUT 46.69,71.37 46.69,68.63 48.82,66.5 R105.P$1 | JP13.1 42.72,17.73 42.72,22.61 JP12.1 43.03,22.91 43.03,36.63 | 43.03,36.63 49.12,36.63 D15.C | 43.03,36.63 38.76,40.89 D17.A
  Bottom 0.356: 37.54,41.81 38.46,40.89 D17.A | 37.54,41.81 33.88,45.47 32.36,45.47 C29.1 | 37.54,41.81 40.28,44.55 40.28,55.83 48.82,64.36 48.82,66.19 R105.P$1
N$157
  Top 0.356: TL274-7.1 338.07,60.71 340.51,60.71 TL274-7.2 340.82,60.4 344.17,57.05 356.97,57.05 R107.P$1 357.28,57.05 357.28,61.32 R106.P$1
N$158
  Bottom 0.356: TL274-7.5 348.13,60.71 342.65,66.19 328.02,66.19 324.97,69.24 324.97,69.55 321.92,72.59 RV2.P$2
N$159
  Bottom 0.356: LED1.A 50.34,23.22 50.34,35.71 50.65,36.02 50.65,60.71 49.12,62.23 R104.P$2
N$160
  Top 0.356: TL274-7.6 350.88,60.71 353.01,60.71 TL274-7.7 353.31,60.71 353.31,61.93 356.97,65.58 R109.P$1 357.28,65.89 357.28,69.55 R108.P$1
N$161
  Bottom 0.356: TL274-7.10 348.13,68.33 345.08,71.37 338.38,71.37 337.16,72.59 RV3.P$2
N$162
  Top 0.356: TL274-7.9 350.88,68.33 353.01,68.33 TL274-7.8 353.31,68.33 353.31,69.24 356.06,71.98 356.06,77.47 353.01,80.52 353.01,96.06 R110.P$1 353.01,96.37 356.36,96.37 R111.P$1
N$163
  Top 0.356: TL274-7.12 343.26,68.33 346.3,71.37 350.88,71.37 352.09,72.59 RV4.P$2
N$164
  Top 0.356: TL274-7.14 338.07,68.33 340.51,68.33 TL274-7.13 340.82,68.33 340.82,76.25 345.08,80.52 345.08,89.66 R113.P$1 345.39,89.97 348.13,89.97 R112.P$1
N$165
  Top 0.356: JP14.1 368.25,90.27 370.99,87.53 370.99,64.97 367.64,61.62 R106.P$2
N$166
  Bottom 0.356: JP14.2 367.94,87.83 368.55,87.83 370.99,85.39 370.99,60.4 367.64,57.05 R107.P$2
N$167
  Top 0.356: JP14.3 370.38,83.26 370.38,72.59 367.64,69.85 R108.P$2
N$168
  Bottom 0.356: JP14.4 367.94,82.65 368.55,82.65 370.38,80.82 370.38,68.63 367.64,65.89 R109.P$2
N$169
  Bottom 0.356: JP14.5 367.94,80.52 359.71,80.52 344.17,96.06 342.65,96.06 R110.P$2
N$170
  Top 0.356: JP14.6 367.64,78.08 365.81,79.91 365.81,95.15 366.72,96.06 R111.P$2
N$171
  Top 0.356: JP14.7 367.94,75.34 366.72,76.56 366.42,76.56 358.8,84.18 358.8,89.66 R112.P$2
N$172
  Bottom 0.356: JP14.8 367.64,72.9 357.28,72.9 340.51,89.66 335.03,89.66 R113.P$2
N$173
  Top 0.356: C30.1 354.23,38.76 354.23,40.89 RV5.P$2 353.92,40.89 351.79,40.89 RV5.P$1 351.48,41.2 349.05,41.2 335.03,55.22 333.81,55.22 322.22,43.64 TL274-8.2 322.22,43.33 318.26,43.33 317.96,43.03 | R130.P$2 317.96,49.12 317.96,46.38 R117.P$2 317.96,46.08 317.96,43.03 | R115.P$2 317.96,39.98 317.96,42.72 R116.P$2 317.96,43.03
N$174
  Top 0.356: C30.2 356.67,38.76 356.67,40.89 RV5.P$3
  Bottom 0.356: TL274-8.1 322.53,46.08 324.97,46.08 328.62,42.42 333.5,42.42 334.42,41.5 334.72,41.5 342.95,33.27 342.95,30.53 344.47,29.01 R118.P$1 344.78,28.7 344.78,28.09 346.61,26.26 353.62,26.26 358.5,31.14 359.71,31.14 361.24,32.66 361.24,34.19 360.63,34.8 360.32,34.8 356.67,38.46 C30.2
N$175
  Top 0.356: JP15.4 302.41,39.98 307.59,39.98 R115.P$1
N$176
  Top 0.356: JP15.3 302.72,42.42 307.29,42.42 307.59,42.72 R116.P$1
N$177
  Top 0.356: JP15.2 302.41,44.86 306.38,44.86 307.59,46.08 R117.P$1
N$178
  Bottom 0.356: 332.89,29.01 334.11,29.01 R118.P$2 | 332.89,29.01 329.23,29.01 324.97,33.27 322.53,33.27 TL274-8.6 | 332.89,29.01 332.89,33.88 334.11,35.1 334.11,37.85 R119.P$1
N$179
  Top 0.356: R140.P$1 360.02,25.96 360.02,29.31 R129.P$1 359.71,29.62 351.48,29.62 347.22,33.88 R128.P$1 346.91,33.88 346.61,33.58 344.78,33.58 | 344.78,33.58 344.78,37.85 R119.P$2 | 344.78,33.58 R120.P$2
N$180
  Top 0.356: TL274-8.7 322.53,31.14 327.71,31.14 328.62,32.05 332.89,32.05 334.11,33.27 R120.P$1
N$181
  Top 0.356: R121.P$2 308.51,69.24 308.51,71.68 309.42,72.59 RV1.P$3
N$182
  Top 0.356: R114.P$1 304.55,65.89 303.02,67.41 303.02,71.07 304.55,72.59 RV1.P$1
N$183
  Top 0.356: R122.P$1 312.17,69.24 314.3,69.24 317.65,72.59 319.18,72.59 RV2.P$1
N$184
  Top 0.356: R123.P$1 319.79,69.24 321.92,69.24 324.05,71.37 326.8,71.37 328.02,72.59 334.42,72.59 RV3.P$1
N$185
  Bottom 0.356: R124.P$1 327.41,69.24 328.02,69.24 333.81,75.03 347.52,75.03 349.66,72.9 RV4.P$1
N$186
  Bottom 0.356: R125.P$2 331.37,69.24 331.37,71.68 334.11,74.42 346,74.42 349.05,71.37 353.31,71.37 354.53,72.59 RV4.P$3
N$187
  Top 0.356: R126.P$2 323.75,69.24 325.58,69.24 327.71,71.37 338.07,71.37 339.29,72.59 RV3.P$3
N$188
  Top 0.356: R127.P$2 316.13,69.24 317.96,69.24 320.09,71.37 322.83,71.37 324.05,72.59 RV2.P$3
N$189
  Top 0.356: R128.P$2 357.28,34.19 357.28,37.24 362.15,42.11 362.15,50.65 363.68,52.17 U1.TIP
N$190
  Top 0.356: R129.P$2 369.77,29.62 369.77,31.45 363.98,37.24 363.98,42.11 U1.RING
N$191
  Top 0.356: JP15.1 302.72,47.6 306.07,47.6 307.59,49.12 R130.P$1
N$192
  Top 0.356: TL274-8.9 329.84,33.27 324.66,33.27 323.44,32.05 318.87,32.05 317.96,31.14 R139.P$2 317.96,30.84 317.96,27.79 R133.P$2 317.96,27.48 317.96,24.74 R132.P$2 317.96,24.43 317.96,21.39 R131.P$2 317.96,21.08 338.38,21.08 338.68,20.78 C31.1 338.99,20.47 339.6,20.47 349.35,10.72 351.48,10.72 RV6.P$1 351.79,10.41 353.92,10.41 RV6.P$2
N$193
  Top 0.356: TL274-8.8 330.15,30.84 330.15,28.7 334.11,24.74 R134.P$1 334.42,24.43 337.46,24.43 341.12,20.78 C31.2 341.43,20.47 346.61,15.29 351.79,15.29 356.36,10.72 RV6.P$3
N$194
  Top 0.356: JP16.4 302.41,21.69 307.29,21.69 307.59,21.39 R131.P$1
N$195
  Top 0.356: JP16.3 302.72,24.74 307.59,24.74 R132.P$1
N$196
  Top 0.356: JP16.2 302.41,27.18 307.29,27.18 307.59,27.48 R133.P$1
N$197
  Top 0.356: R135.P$1 334.11,48.51 334.11,47.6 330.15,43.64 TL274-8.13 330.15,43.33 331.98,41.5 331.98,38.15 344.47,25.65 344.47,24.74 R134.P$2
N$198
  Top 0.356: R136.P$2 344.78,53.7 344.78,48.82 R135.P$2
  Bottom 0.356: R135.P$2 344.78,48.51 344.78,43.64 R137.P$1 344.78,43.33 344.78,39.68 348.74,35.71 348.74,28.09 | 348.74,28.09 354.53,28.09 359.71,33.27 R138.P$1 | 348.74,28.09 347.22,28.09 R141.P$1
N$199
  Top 0.356: TL274-8.14 330.15,46.38 330.15,49.73 334.11,53.7 R136.P$1
N$200
  Top 0.356: R137.P$2 334.42,43.33 342.65,43.33 354.84,31.14 360.32,31.14 363.68,27.79 363.68,22 U2.TIP
N$201
  Bottom 0.356: R138.P$2 369.77,33.27 369.77,31.45 365.51,27.18 365.51,13.46 363.98,11.94 U2.RING
N$202
  Top 0.356: JP16.1 302.72,29.62 306.38,29.62 307.59,30.84 R139.P$1
N$203
  Top 0.356: TL274-9.3 323.75,14.07 325.58,12.24 325.58,11.33 323.75,9.5 TL274-9.5 323.44,9.5 323.14,9.8 302.72,9.8 SPLIT1_IN.1
N$204
  Top 0.356: TL274-9.1 323.75,19.25 323.75,17.12 TL274-9.2 323.75,16.81 324.97,15.6 332.59,15.6 333.5,14.68 337.77,14.68 JP18.1
N$205
  Top 0.356: TL274-9.10 331.37,9.5 333.2,11.33 333.2,12.24 331.37,14.07 TL274-9.12
  Bottom 0.356: SPLIT2_IN.1 302.72,3.71 317.96,3.71 322.22,7.98 329.84,7.98 331.06,9.2 TL274-9.10
N$206
  Top 0.356: 331.37,5.84 331.37,6.45 TL274-9.9 | 331.37,5.84 331.37,4.32 TL274-9.8 | 331.37,5.84 337.77,5.84 JP17.1
N$207
  Top 0.356: TL274-9.7 323.75,4.32 323.75,6.45 TL274-9.6 323.75,6.76 324.97,7.98 332.28,7.98 335.94,11.63 337.77,11.63 JP18.2
N$208
  Top 0.356: TL274-9.13 331.37,17.12 331.37,19.25 TL274-9.14
  Bottom 0.356: JP17.2 333.2,7.67 333.2,14.99 331.37,16.81 TL274-9.13
N$209
  Top 0.356: R141.P$2 357.58,27.79 357.58,21.39 362.15,16.81 362.15,11.02 365.81,7.37 369.47,7.37 JP20.1
N$210
  Top 0.356: JP19.1 369.77,37.85 369.77,35.71 371.6,33.88 371.6,27.48 370.08,25.96 R140.P$2
VDD  (via drill 0.51)
  Top 0.356: R124.P$2 327.41,58.88 325.58,58.88 324.05,60.4 321.31,60.4 319.79,58.88 R123.P$2 | R114.P$2 304.55,66.8 312.17,59.18 R122.P$2 | TL274-5.4 244.5,64.36 239.93,59.79 239.93,57.96 239.62,57.66 R68.P$2 | R63.P$2 228.96,92.1 228.96,88.75 R65.P$2 228.96,88.44 229.87,87.53 229.87,85.39 R67.P$2 229.87,85.09 228.04,85.09 224.99,82.04 217.68,82.04 209.45,73.81 | 555.8 252.43,86.31 259.13,86.31 261.26,88.44 273.46,88.44 R79.P$2 | R79.P$2 273.76,88.44 273.76,85.39 R81.P$2 273.76,85.09 275.28,83.57 275.28,81.13 274.68,80.52 274.68,69.85 275.59,68.94 276.81,68.94 284.12,61.62 284.12,56.44 R82.P$2 | R77.P$2 273.76,92.1 273.76,88.75 R79.P$2 | TL274.4 68.02,43.33 58.57,52.78 58.57,54.91 56.44,57.05 JP3.3 | v111.61,42.11 111.61,44.55 114.05,46.99 116.48,46.99 117.09,47.6 117.09,49.73 122.28,54.91 R32.P$2 | 170.74,85.09 169.82,86 165.86,86 164.34,84.48 160.38,84.48 159.77,83.87 159.77,80.21 161.59,78.38 LM13700.11 | 170.74,85.09 170.74,77.77 165.25,72.29 R60.P$1 | TL274-6.4 185.37,72.59 190.86,78.08 190.86,80.52 192.38,82.04 193.6,82.04 196.34,84.78 196.34,87.22 THAT2180.7 | 170.74,85.09 175.01,89.36 178.05,89.36 181.71,93.02 194.51,93.02 196.04,91.49 R98.P$2 | 209.45,73.81 209.45,43.94 216.15,37.24 216.15,16.51 S1.3 | 209.45,73.81 207.31,75.95 DUALOPAMP.8
  Bottom 0.356: R82.P$2 284.43,56.44 284.43,60.1 288.7,64.36 TL274-1.4 289,64.67 291.74,64.67 295.4,68.33 297.54,68.33 301.5,72.29 | 301.5,72.29 304.55,69.24 R114.P$2 | 301.5,72.29 299.67,74.12 299.67,82.96 296.62,86 555-1.8 | TL274-7.4 345.39,60.71 343.56,62.54 331.06,62.54 327.41,58.88 R124.P$2 | R123.P$2 319.79,57.35 | 319.79,57.35 319.79,41.2 322.22,38.76 TL274-8.4 322.22,38.46 320.4,36.63 320.4,14.99 323.44,11.94 TL274-9.4 | 319.79,57.35 315.21,57.35 314,58.57 312.17,58.57 R122.P$2 | R65.P$2 228.96,88.75 236.88,88.75 238.4,90.27 248.16,90.27 252.12,86.31 555.8 252.12,86 249.68,83.57 249.68,69.55 244.81,64.67 TL274-5.4 | R9.P$2 82.65,55.22 82.65,56.13 80.82,57.96 80.82,59.79 83.87,62.84 83.87,63.75 78.08,69.55 74.73,69.55 73.81,70.46 73.81,81.13 75.64,82.96 TL274-2.4 75.95,82.96 80.82,82.96 82.65,81.13 R14.P$1 82.96,81.13 84.48,82.65 84.48,87.83 | 84.48,87.83 80.21,92.1 74.42,92.1 69.24,86.92 66.8,86.92 63.14,83.26 63.14,73.81 56.44,67.11 56.44,57.05 JP3.3 | v111.61,42.11 110.39,42.11 109.47,43.03 107.64,43.03 TL274-3.4 | S1.3 216.46,16.2 219.2,16.2 227.43,7.98 252.73,7.98 260.96,16.2 S2.3 | 198.48,89.36 199.7,89.36 203.35,85.7 203.35,81.13 207.01,77.47 207.01,76.25 DUALOPAMP.8 | 198.48,89.36 196.65,87.53 THAT2180.7 | 198.48,89.36 198.17,89.36 196.34,91.19 R98.P$2 | R60.P$1 164.95,71.98 163.42,71.98 153.98,62.54 137.82,62.54 130.5,55.22 122.58,55.22 R32.P$2 122.28,55.22 120.45,57.05 120.45,58.88 123.19,61.62 123.19,63.75 117.4,69.55 114.05,69.55 113.13,70.46 113.13,81.13 114.96,82.96 TL274-4.4 115.27,82.96 120.45,82.96 122.28,81.13 R37.P$1 122.58,81.13 123.8,82.35 123.8,87.83 119.53,92.1 90.58,92.1 86.31,87.83 84.48,87.83
VNEG  (via drill 0.51)
  Top 0.356: TL274-7.11 345.39,68.02 339.9,62.54 335.03,62.54 331.37,58.88 R125.P$1 331.06,58.57 329.23,58.57 328.02,57.35 324.97,57.35 323.75,58.57 R126.P$1 323.44,58.57 322.22,57.35 319.18,57.35 317.96,58.57 316.13,58.57 R127.P$1 315.82,58.57 314.6,57.35 311.56,57.35 310.34,58.57 308.51,58.57 R121.P$1 | v73.51,48.21 73.51,46.99 | 73.51,46.99 73.51,45.47 75.64,43.33 TL274.11 | JP3.1 56.13,51.87 54,54 54,57.35 54.91,58.27 60.1,58.27 62.54,55.83 R23.P$1 | 73.51,46.99 76.86,46.99 77.77,47.9 77.77,49.73 81.43,53.39 83.26,53.39 84.48,52.17 84.48,48.21 92.41,40.28 93.93,40.28 95.15,41.5 95.15,48.21 101.85,54.91 101.85,55.52 R46.P$1 | 148.49,77.16 149.1,77.77 R50.P$1 | 148.49,77.16 147.88,76.56 147.88,73.81 149.1,72.59 149.1,71.37 R52.P$1 | DUALOPAMP.4 199.7,68.63 200.91,69.85 200.91,76.86 200.3,77.47 198.78,77.47 193.9,72.59 192.99,72.59 TL274-6.11 192.68,72.29 191.47,71.07 184.15,71.07 180.8,67.72 162.51,67.72 160.99,66.19 152.76,66.19 R59.P$1 | 148.49,77.16 139.65,86 121.67,86 120.75,86.92 114.05,86.92 108.86,92.1 100.02,92.1 99.11,91.19 99.11,89.36 105.21,83.26 107.34,83.26 TL274-4.11
  Bottom 0.356: 302.72,64.36 296.62,64.36 TL274-1.11 | 302.72,64.36 308.2,58.88 R121.P$1 | R126.P$1 323.44,58.57 320.4,55.52 320.4,45.47 321,44.86 323.75,44.86 329.84,38.76 TL274-8.11 330.15,38.76 330.76,39.37 335.03,39.37 335.94,38.46 335.94,28.4 329.23,21.69 329.23,13.77 331.06,11.94 TL274-9.11 | TL274-3.11 114.96,43.33 110.08,43.33 108.86,44.55 106.43,44.55 103.38,47.6 103.38,54.3 102.16,55.52 R46.P$1 102.16,55.83 103.99,57.66 103.99,68.94 103.68,69.24 103.68,74.12 105.51,75.95 105.51,81.13 107.34,82.96 TL274-4.11 | v73.51,48.21 67.41,54.3 64.06,54.3 62.84,55.52 R23.P$1 62.84,55.83 64.67,57.66 64.67,68.94 64.36,69.24 64.36,74.12 65.89,75.64 65.89,80.82 68.02,82.96 TL274-2.11 | LM13700.6 154.28,78.08 156.11,76.25 156.11,69.55 152.76,66.19 R59.P$1 152.45,66.19 148.49,66.19 147.88,66.8 147.88,68.33 149.1,69.55 149.1,71.07 R52.P$1 | 254.25,95.76 254.25,66.5 252.43,64.67 TL274-5.11 | 254.25,95.76 252.43,97.59 198.78,97.59 192.68,91.49 R101.P$1 192.38,91.19 190.25,89.05 190.25,86 190.55,85.7 190.55,74.73 192.68,72.59 TL274-6.11 | 302.72,64.36 302.72,64.97 306.07,68.33 306.07,69.55 304.24,71.37 303.94,71.37 300.28,75.03 300.28,94.54 296.62,98.2 256.69,98.2 254.25,95.76

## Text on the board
tNames: PWR | VCO1 | VCO2 | VCF | VCA | ADSR1 | ADSR2 | OPS | cv1-1 | CONST CV | cv1-2 | cv2-1 | A | A | cv2-2 | cv3-1 | cv3-2 | cv4-1 | cv4-2 | D | D | + | IN | MOD | OUT | audio | cutoff cv 1 | bandpass | S | S | cutoff cv 2 | lowpass | MIX1 | mix in | - | CUT / OFF | RES / ONA / NCE | R | R | mix 1 out | IN | OUT | audio | audio | MIX2 | mix in | cv1 | OUT | cv2 | IN | MOD | IN | MOD | IN | OUT | IN | OUT | trigger | cv1 | trigger | cv1 | 1v/oct | linfm | 1v/oct | linfm | + | - | cv2 | cv2 | 1v/oct | hard sync | 1v/oct | hard sync | split1 out | 1v/oct | pwm ctrl | 1v/oct | pwm ctrl | cv3 | cv3 | SPLIT | coarse | coarse | fine | fine | OUT | OUT | umodular / v 2016.01 / sinneb@gmail.com | split2 out | mix 2 out | saw | saw | pulse | pulse
200bmp: /Users/Arthur/Desktop/Untitled-1.bmp | /Users/Arthur/Desktop/Untitled-1.bmp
